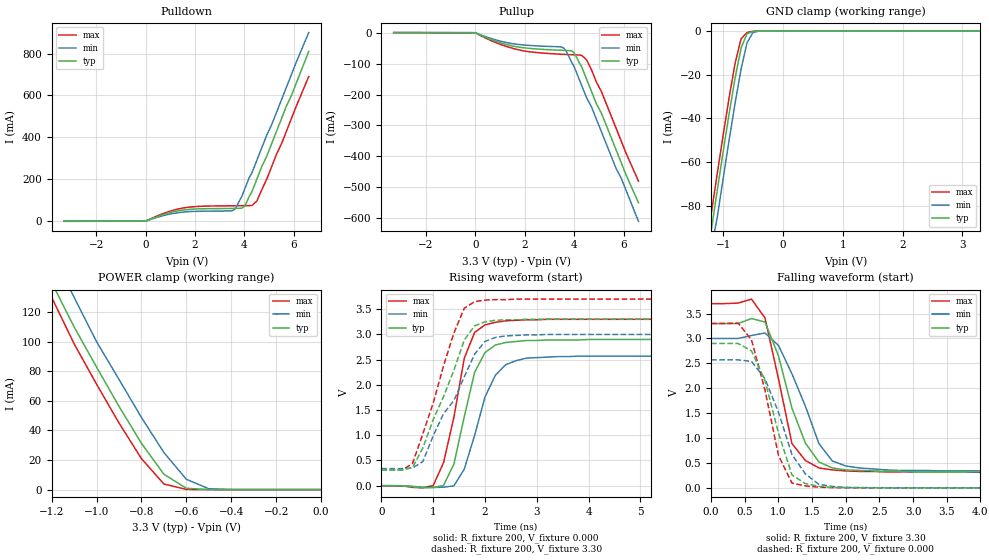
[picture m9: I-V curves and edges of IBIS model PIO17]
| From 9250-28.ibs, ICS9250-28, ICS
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|   Model PIO17
[Model]   PIO17
Model_type   I/O
Polarity   Non-Inverting
Enable   Active-High
Vinl =   0.80V
Vinh =   2.00V
Vmeas =   1.50V
Cref =  20.00pF
Rref =  0.000
Vref =   1.50V
C_comp   5.50pF   5.00pF   6.00pF
[Temperature Range]   27.00   70.00   0.000
[Voltage Range]   3.30V   3.00V   3.70V
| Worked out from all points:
|   slope of the pulldown table from 0 to 0.495 V, typ, clamps not added: 21.7 ohm
|   slope of the pullup table from 0 to 0.495 V, typ, clamps not added: 28.3 ohm
|   GND clamp passes 1 mA (typ) near -0.57 V on its own axis
|   POWER clamp passes 1 mA (typ) near -0.60 V on its own axis
|   rising waveform, R_fixture 200, V_fixture 0.000: 20-80 % time 404ps typ, 483ps min, 399ps max; typ from 0 V to 2.9 V
|   rising waveform, R_fixture 200, V_fixture 3.30: 20-80 % time 681ps typ, 783ps min, 612ps max; typ from 0.31 V to 3.3 V
|   falling waveform, R_fixture 200, V_fixture 3.30: 20-80 % time 413ps typ, 473ps min, 321ps max; typ from 3.3 V to 0.31 V
|   falling waveform, R_fixture 200, V_fixture 0.000: 20-80 % time 380ps typ, 440ps min, 333ps max; typ from 2.9 V to 0 V
[Pulldown]
| voltage   I(typ)   I(min)   I(max)
-3.3V     -500uA     -400uA     -600uA
0V        0A         0A         -49.56pA
1.5V      52.87mA    43.05mA    62.51mA
3.6V      60.87mA    56.04mA    73.58mA
3.9V      62.15mA    120mA      73.97mA
4V        71.8mA     150mA      74.1mA
4.3V      140mA      230mA      74.63mA
4.5V      200mA      290mA      95.69mA
4.9V      310mA      410mA      200mA
5.1V      370mA      460mA      260mA
6.1V      660mA      760mA      550mA
6.6V      810mA      900mA      690mA
[Pullup]
| voltage   I(typ)   I(min)   I(max)
-3.3V     400uA      300uA      500uA
0V        270pA      -3.2pA     920pA
1.7V      -45.75mA   -37.5mA    -54.3mA
3.6V      -57.07mA   -51.21mA   -70.09mA
4V        -65.81mA   -110mA     -71.4mA
4.3V      -110mA     -170mA     -72.92mA
4.5V      -150mA     -210mA     -87.44mA
4.7V      -190mA     -240mA     -120mA
5.1V      -260mA     -320mA     -190mA
5.7V      -380mA     -440mA     -310mA
6.1V      -460mA     -510mA     -390mA
6.6V      -550mA     -610mA     -480mA
[GND_clamp]
| voltage   I(typ)   I(min)   I(max)
-3.3V     -490mA     -500mA     -480mA
-1.3V     -110mA     -120mA     -100mA
-1.2V     -91.53mA   -100mA     -83.86mA
-1.1V     -73.3mA    -85.6mA    -65.64mA
-1V       -55.38mA   -67.61mA   -47.78mA
-900mV    -37.97mA   -50mA      -30.57mA
-800mV    -21.59mA   -33.06mA   -14.82mA
-700mV    -7.85mA    -17.49mA   -3.64mA
-600mV    -1.29mA    -5.41mA    -750uA
-500mV    -280uA     -750uA     -190uA
-400mV    -52.44uA   -130uA     -25.65uA
3.3V      58.7pA     940nA      23.35pA
[POWER_clamp]
| voltage   I(typ)   I(min)   I(max)
-3.3V     740mA      760mA      730mA
-1.2V     140mA      160mA      130mA
-1.1V     110mA      130mA      98.55mA
-1V       82.82mA    100mA      71.28mA
-900mV    56.3mA     74.52mA    45.03mA
-800mV    31.29mA    48.77mA    20.93mA
-700mV    10.41mA    25.08mA    3.78mA
-600mV    890uA      7mA        140uA
-500mV    29.3uA     580uA      2.74uA
-400mV    680nA      26.19uA    43.51nA
0V        58.7pA     690pA      33.79pA
[Ramp]
| variable   typ   min   max
dV/dt_r   1.74/0.38n   1.54/0.46n   1.98/0.34n
dV/dt_f   1.79/0.35n   1.60/0.41n   2.03/0.31n
R_load = 200
[Rising Waveform]
R_fixture = 200
V_fixture = 0.000
V_fixture_min = 0.000
V_fixture_max = 0.000
| time   V(typ)   V(min)   V(max)
0s        0V         0V         0V
1ns       -34.95mV   -35.15mV   2.23mV
1.2ns     5.53mV     -29.6mV    460mV
1.4ns     430mV      -2.25mV    1.36V
1.6ns     1.37V      330mV      2.53V
1.8ns     2.25V      1V         3.04V
2ns       2.64V      1.76V      3.19V
2.4ns     2.84V      2.4V       3.27V
2.8ns     2.88V      2.53V      3.29V
10ns      2.9V       2.57V      3.3V
[Rising Waveform]
R_fixture = 200
V_fixture = 3.30
V_fixture_min = 3.00
V_fixture_max = 3.70
| time   V(typ)   V(min)   V(max)
0s        310mV      340mV      310mV
600ps     360mV      350mV      440mV
800ps     750mV      480mV      1.03V
1.2ns     1.77V      1.43V      2.38V
1.4ns     2.29V      1.69V      3.03V
1.6ns     2.89V      2.16V      3.52V
1.8ns     3.17V      2.61V      3.65V
2.2ns     3.28V      2.94V      3.69V
2.8ns     3.3V       2.99V      3.7V
10ns      3.3V       3V         3.7V
[Falling Waveform]
R_fixture = 200
V_fixture = 3.30
V_fixture_min = 3.00
V_fixture_max = 3.70
| time   V(typ)   V(min)   V(max)
0s        3.3V       3V         3.7V
600ps     3.4V       3.06V      3.79V
800ps     3.33V      3.11V      3.41V
1ns       2.65V      2.86V      2.19V
1.2ns     1.6V       2.29V      890mV
1.4ns     900mV      1.64V      550mV
1.6ns     520mV      890mV      400mV
1.8ns     400mV      540mV      360mV
2.6ns     330mV      360mV      320mV
10ns      310mV      340mV      310mV
[Falling Waveform]
R_fixture = 200
V_fixture = 0.000
V_fixture_min = 0.000
V_fixture_max = 0.000
| time   V(typ)   V(min)   V(max)
0s        2.9V       2.57V      3.3V
400ps     2.9V       2.57V      3.31V
600ps     2.75V      2.54V      2.97V
800ps     2.15V      2.19V      1.96V
1ns       1.1V       1.52V      650mV
1.2ns     260mV      670mV      96.46mV
1.4ns     84.47mV    280mV      38.92mV
1.6ns     29.21mV    69.97mV    12.81mV
2ns       5.24mV     8.4mV      3.33mV
10ns      0V         0V         6.59uV
